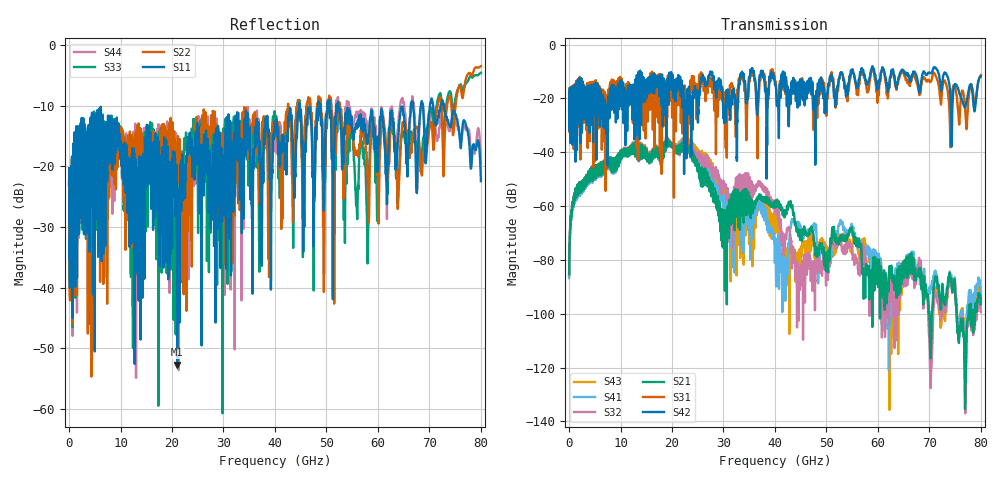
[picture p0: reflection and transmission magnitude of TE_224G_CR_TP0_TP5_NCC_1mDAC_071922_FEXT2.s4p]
!! Reference: tracy_3df_01a_2207
!! CHANNEL DESCRIPTION: TP0_TP5 CR Channel using 1meter DAC, CABLED NCC Host
!! MODEL DESCRIPTION: s4p, FEXT2
!! CONNECTOR DESCRIPTION: OSFP 200G OTB, NCC Socket
!! CABLE DESCRIPTION: 1meter 26AWG Cable
!! MODEL STATUS: Developmental
!! PORT DEFINITIONS:
!! Port  1  ----->  Side A  Side B  <-----  Port  2
!! Port  3  ----->  Side A  Side B  <-----  Port  4
# GHz S MA R 50
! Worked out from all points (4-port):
!   8000 points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, 10 MHz to 80 GHz, reference 50 ohm
!   strongest paths, dB at 10 MHz, 20.01 GHz, 40.01 GHz, 60.01 GHz, 80 GHz:
!     S42: -24.5, -15.5, -14.9, -14.2, -11.8
!     S31: -24.5, -26.1, -13.7, -17.6, -11.4
!     S21: -85.3, -37.4, -60.3, -88.8, -96.6
!     S32: -85.6, -37.3, -61.8, -86.3, -99.4
!     S41: -86.8, -37.0, -75.0, -84.4, -91.8
!     S43: -86.1, -36.5, -69.0, -83.0, -94.7
!   lowest |S11| = -52.7 dB at 21.01 GHz (marker M1), VSWR 1.00, Z = 50 + j0.231 ohm
!   |S11| at or under -10 dB: start of sweep to 44.68 GHz; 52.32 GHz to 66.38 GHz (14.06 GHz wide, 23.7 % of centre); 72.83 GHz to end of sweep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
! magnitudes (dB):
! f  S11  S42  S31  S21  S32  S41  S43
! 10 MHz  -23.1  -24.5  -24.5  -85.3  -85.6  -86.8  -86.1
! 4.04 GHz  -19.6  -18.9  -21.2  -46.6  -46.6  -47.0  -46.6
! 21.01 GHz  -52.7  -15.9  -17.3  -37.8  -37.2  -38.0  -37.0
! 29.93 GHz  -20.8  -24.0  -17.7  -73.6  -52.1  -59.8  -57.1
! 41.47 GHz  -16.0  -11.4  -13.5  -62.3  -71.4  -82.5  -74.1
! 43.55 GHz  -18.8  -12.4  -12.4  -63.2  -78.1  -65.6  -76.9
! 80 GHz  -22.4  -11.8  -11.4  -96.6  -99.4  -91.8  -94.7
